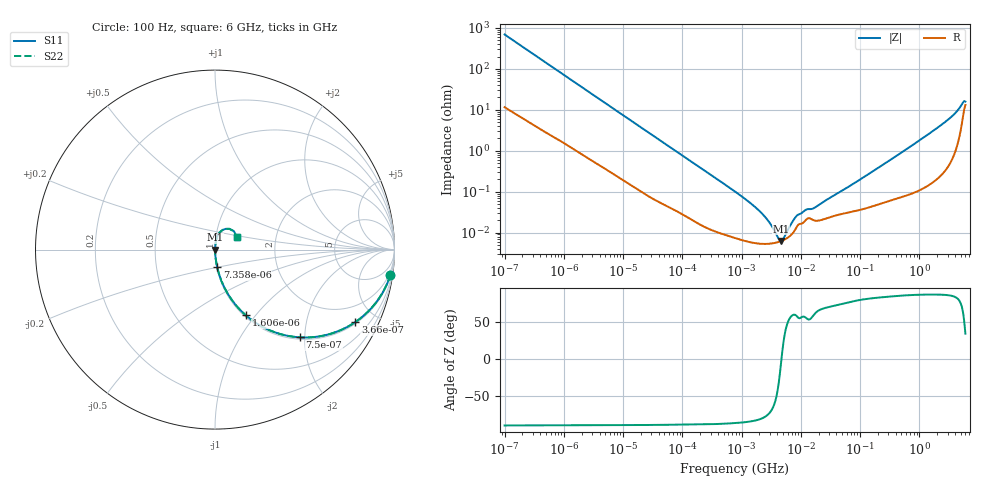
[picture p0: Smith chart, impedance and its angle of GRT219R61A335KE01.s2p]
!Murata Part Number: GRT219R61A335KE01
!These Parameters are Measured in Series Mode Connection
!Data Generated on Jun 19, 2026
!  o--ll--o
!Port1  Port2
!  o------o
!Operation Temp=25[degC], DC Bias Voltage=0[V]
!Freq. Start=100[Hz] Stop=6[GHz] 401[Steps]
# Hz S RI R 50
!Freq.(Hz) S11(Real) S11(Imag) S21(Real) S21(Imag) S12(Real) S12(Imag) S22(Real) S22(Imag)
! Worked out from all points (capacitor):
!   401 points, 100 Hz to 6 GHz, reference 50 ohm
!   read as one part in series: C = 2.29 uF near 109 Hz
!   lowest |Z| = 6.21 mohm at 4.644 MHz (marker M1)
!   series resonance near 4.713 MHz, so ESL is about 500 pH
!   S11 on the Smith chart (normalised r, x): 100 Hz: 1, -14; 366 Hz: 1.07, -3.83; 750 Hz: 1.04, -1.89; 1.606 kHz: 1.02, -0.89; 7.358 kHz: 1.01, -0.20; 6 GHz: 1.26, +0.18
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100  0.9773 -0.1408  0.0227 0.1408  0.0227 0.1408  0.9773 -0.1408
205  0.9167 -0.2675  0.0833 0.2675  0.0833 0.2675  0.9167 -0.2675
366  0.7818 -0.4037  0.2182 0.4037  0.2182 0.4037  0.7818 -0.4037
750  0.4723 -0.4889  0.5277 0.4889  0.5277 0.4889  0.4723 -0.4889
1606  0.1715 -0.366  0.8285 0.366  0.8285 0.366  0.1715 -0.366
2008  0.119 -0.3127  0.881 0.3127  0.881 0.3127  0.119 -0.3127
7358  0.0123 -0.0981  0.9877 0.0981  0.9877 0.0981  0.0123 -0.0981
40335  0.000904 -0.0186  0.9991 0.0186  0.9991 0.0186  0.000904 -0.0186
774597  7.46e-05 -0.001  0.9999 0.001  0.9999 0.001  7.46e-05 -0.001
2074311  5.34e-05 -0.000317  0.9999 0.000317  0.9999 0.000317  5.34e-05 -0.000317
2713602  5.31e-05 -0.000201  0.9999 0.000201  0.9999 0.000201  5.31e-05 -0.000201
3712478  5.62e-05 -8.38e-05  0.9999 8.38e-05  0.9999 8.38e-05  5.62e-05 -8.38e-05
4643984  6.19e-05 -5.1e-06  0.9999 5.1e-06  0.9999 5.1e-06  6.19e-05 -5.1e-06
5809218  7.26e-05 7.44e-05  0.9999 -7.44e-05  0.9999 -7.44e-05  7.26e-05 7.44e-05
8692127  0.000143 0.000222  0.9999 -0.000222  0.9999 -0.000222  0.000143 0.000222
1.243624e7  0.00021 0.0003  0.9998 -0.0003  0.9998 -0.0003  0.00021 0.0003
1.555665e7  0.000208 0.000318  0.9998 -0.000318  0.9998 -0.000318  0.000208 0.000318
3.124326e8  0.000629 0.00572  0.9994 -0.00572  0.9994 -0.00572  0.000629 0.00572
2.450438e9  0.00465 0.0442  0.9954 -0.0442  0.9954 -0.0442  0.00465 0.0442
4.385646e9  0.0219 0.0903  0.9781 -0.0903  0.9781 -0.0903  0.0219 0.0903
5.245841e9  0.0588 0.1155  0.9412 -0.1155  0.9412 -0.1155  0.0588 0.1155
6e9  0.1212 0.0694  0.8788 -0.0694  0.8788 -0.0694  0.1212 0.0694
